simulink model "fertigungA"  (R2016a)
settings: Solver=FixedStepDiscrete  StartTime=0.0  StopTime=25.1  RelTol=1e-3
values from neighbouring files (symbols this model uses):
  dt = block.DialogPrm(4).Data    [sfun_oven.m]
  t0 = block.DialogPrm(5).Data    [sfun_oven.m]
undefined symbols (not defined in the file or in its folder): m0, ndelay
libraries: simulink x1

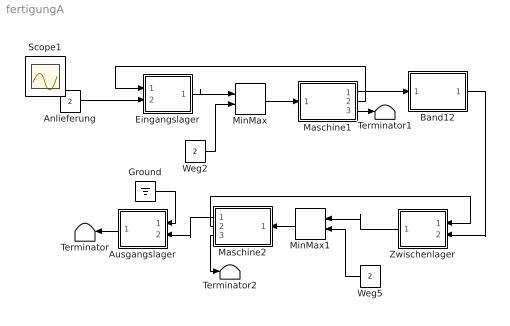
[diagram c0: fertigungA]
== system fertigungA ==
  Anlieferung : Constant  Value=2
  Ausgangslager : Subsystem
  Band12 : Subsystem
  Eingangslager : Subsystem
  Ground : Ground
  Maschine1 : Subsystem
  Maschine2 : Subsystem
  MinMax : MinMax  Inputs=2
  MinMax1 : MinMax  Inputs=2
  Terminator : Terminator
  Terminator1 : Terminator
  Terminator2 : Terminator
  Weg2 : Constant  Value=2
  Weg5 : Constant  Value=2
  Zwischenlager : Subsystem
  Scope1 : Scope
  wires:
  Anlieferung/1 -> Eingangslager/2(In2)
  MinMax/1 -> Maschine1/1(in)
  Eingangslager/1(Out1) -> MinMax/1
  Weg2/1 -> MinMax/2
  Maschine1/1(out) -> Band12/1(In)
  MinMax1/1 -> Maschine2/1(in)
  Weg5/1 -> MinMax1/2
  Maschine2/1(out) -> Ausgangslager/2(In2)
  Maschine1/2(increment) -> Eingangslager/1(In1)
  Ausgangslager/1(Out1) -> Terminator/1
  Maschine1/3(load) -> Terminator1/1
  Zwischenlager/1(Out1) -> MinMax1/1
  Band12/1(Out) -> Zwischenlager/2(In2)
  Maschine2/2(increment) -> Zwischenlager/1(In1)
  Maschine2/3(load) -> Terminator2/1
  Ground/1 -> Ausgangslager/1(In1)

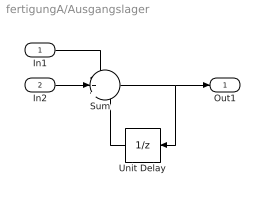
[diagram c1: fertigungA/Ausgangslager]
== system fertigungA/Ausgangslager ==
  In1 : Inport
  In2 : Inport  Port=2
  Sum : Sum  Inputs=-++
  Unit Delay : UnitDelay  InitialCondition=m0  SampleTime=[dt, t0]
  Out1 : Outport
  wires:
  Unit Delay/1 -> Sum/3
  In2/1 -> Sum/2
  Sum/1 -> Unit Delay/1, Out1/1
  In1/1 -> Sum/1

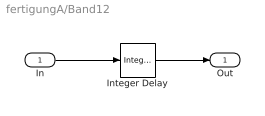
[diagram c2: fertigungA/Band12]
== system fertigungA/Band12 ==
  In : Inport
  Integer Delay : simulink/Discrete/Integer Delay  NumDelays=ndelay  vinit=0.0  samptime=[dt,t0]
  Out : Outport
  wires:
  Integer Delay/1 -> Out/1
  In/1 -> Integer Delay/1

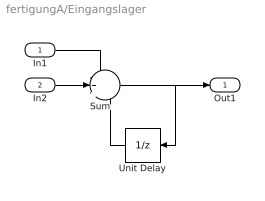
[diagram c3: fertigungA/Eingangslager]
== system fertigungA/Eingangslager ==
  In1 : Inport
  In2 : Inport  Port=2
  Sum : Sum  Inputs=-++
  Unit Delay : UnitDelay  InitialCondition=m0  SampleTime=[dt, t0]
  Out1 : Outport
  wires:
  Unit Delay/1 -> Sum/3
  In2/1 -> Sum/2
  Sum/1 -> Unit Delay/1, Out1/1
  In1/1 -> Sum/1

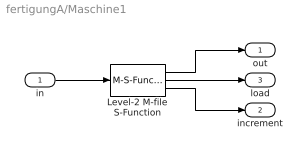
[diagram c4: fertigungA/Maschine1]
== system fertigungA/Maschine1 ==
  in : Inport
  Level-2 M-file S-Function : M-S-Function  FunctionName=sfun_oven  Parameters=capacity, cookingtime, initload, dt, t0
  out : Outport
  increment : Outport  Port=2
  load : Outport  Port=3
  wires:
  Level-2 M-file S-Function/3 -> increment/1
  Level-2 M-file S-Function/2 -> load/1
  Level-2 M-file S-Function/1 -> out/1
  in/1 -> Level-2 M-file S-Function/1

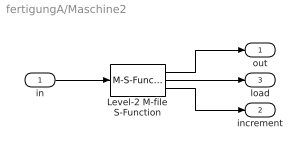
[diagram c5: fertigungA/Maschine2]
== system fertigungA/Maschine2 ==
  in : Inport
  Level-2 M-file S-Function : M-S-Function  FunctionName=sfun_oven  Parameters=capacity, cookingtime, initload, dt, t0
  out : Outport
  increment : Outport  Port=2
  load : Outport  Port=3
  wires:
  Level-2 M-file S-Function/3 -> increment/1
  Level-2 M-file S-Function/2 -> load/1
  Level-2 M-file S-Function/1 -> out/1
  in/1 -> Level-2 M-file S-Function/1

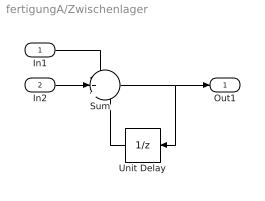
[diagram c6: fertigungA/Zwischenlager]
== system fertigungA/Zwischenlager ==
  In1 : Inport
  In2 : Inport  Port=2
  Sum : Sum  Inputs=-++
  Unit Delay : UnitDelay  InitialCondition=m0  SampleTime=[dt, t0]
  Out1 : Outport
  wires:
  Unit Delay/1 -> Sum/3
  In2/1 -> Sum/2
  Sum/1 -> Unit Delay/1, Out1/1
  In1/1 -> Sum/1
